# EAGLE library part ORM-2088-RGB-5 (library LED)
ORM 2088RGB-5 8x8 LED RGB Matrix
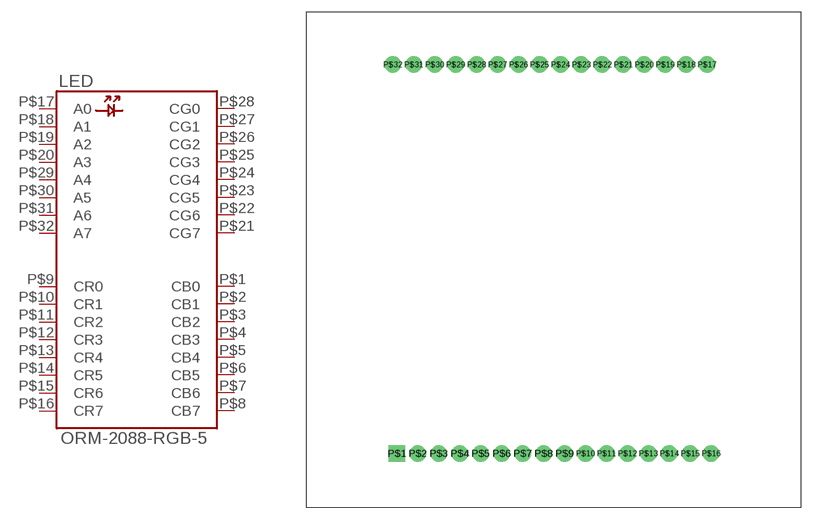
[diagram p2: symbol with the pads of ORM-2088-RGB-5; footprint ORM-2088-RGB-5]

Designator prefix LED

## ORM-2088-RGB-5  [ORM-2088-RGB-5]
P$1  CB0
P$2  CB1
P$3  CB2
P$4  CB3
P$5  CB4
P$6  CB5
P$7  CB6
P$8  CB7
P$9  CR0
P$10  CR1
P$11  CR2
P$12  CR3
P$13  CR4
P$14  CR5
P$15  CR6
P$16  CR7
P$17  A0
P$18  A1
P$19  A2
P$20  A3
P$21  CG7
P$22  CG6
P$23  CG5
P$24  CG4
P$25  CG3
P$26  CG2
P$27  CG1
P$28  CG0
P$29  A4
P$30  A5
P$31  A6
P$32  A7

## Footprint ORM-2088-RGB-5 (pad centres in mm)
drill 0.8 pad 2 square: P$1 -19,-23.5
drill 0.8 pad 2: P$2 -16.46,-23.5; P$3 -13.92,-23.5; P$4 -11.38,-23.5; P$5 -8.84,-23.5; P$6 -6.3,-23.5; P$7 -3.76,-23.5; P$8 -1.22,-23.5; P$9 1.32,-23.5; P$10 3.86,-23.5; P$11 6.4,-23.5; P$12 8.94,-23.5; P$13 11.48,-23.5; P$14 14.02,-23.5; P$15 16.56,-23.5; P$16 19.1,-23.5; P$17 18.6,23.66; P$18 16.06,23.66; P$19 13.52,23.66; P$20 10.98,23.66; P$21 8.44,23.66; P$22 5.9,23.66; P$23 3.36,23.66; P$24 0.82,23.66; P$25 -1.72,23.66; P$26 -4.26,23.66; P$27 -6.8,23.66; P$28 -9.34,23.66; P$29 -11.88,23.66; P$30 -14.42,23.66; P$31 -16.96,23.66; P$32 -19.5,23.66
